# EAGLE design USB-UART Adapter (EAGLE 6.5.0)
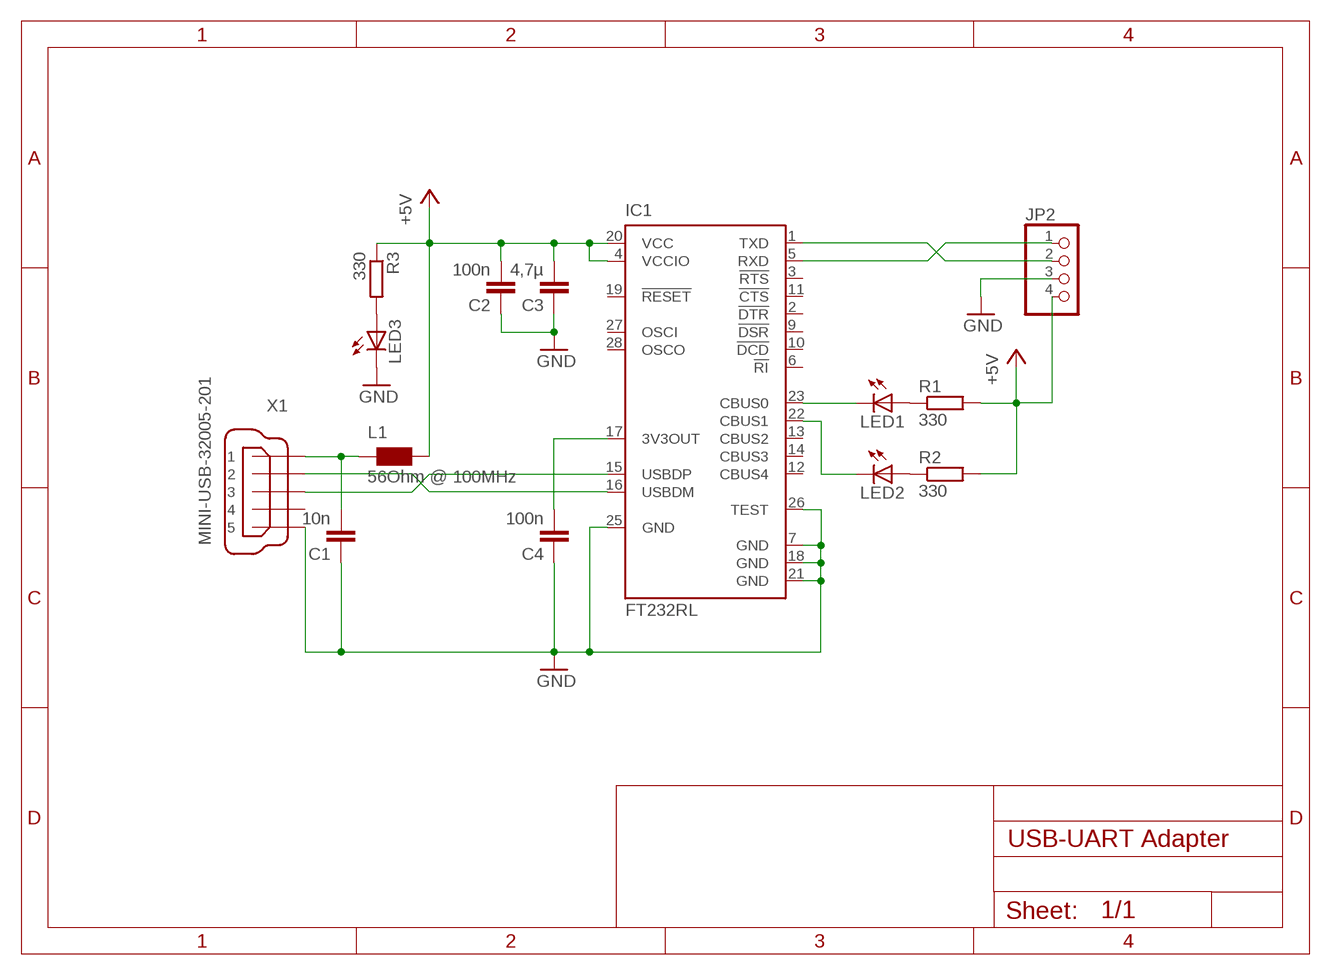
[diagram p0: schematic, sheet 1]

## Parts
C1  10n  C-EUC0805  [C0805]
C2  100n  C-EUC0805  [C0805]
C3  4,7µ  C-EUC0805  [C0805]
C4  100n  C-EUC0805  [C0805]
IC1  FT232RL  [SSOP28]
JP2  PINHD-1X4  [1X04]
L1  56Ohm @ 100MHz  SMD_BEADS_FASTRON_SMB/001  [SMB/001]
LED1  LEDSML0805  [SML0805]
LED2  LEDSML0805  [SML0805]
LED3  LEDSML0805  [SML0805]
R1  330  R-EU_R0805  [R0805]
R2  330  R-EU_R0805  [R0805]
R3  330  R-EU_R0805  [R0805]
X1  MINI-USB-32005-201  [32005-201]

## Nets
+5V: C2.2 C3.2 IC1.4(VCCIO) IC1.20(VCC) JP2.4 L1.2 R1.2 R2.2 R3.1
GND: C1.1 C2.1 C3.1 C4.1 IC1.7(GND) IC1.18(GND) IC1.21(GND) IC1.25(GND) IC1.26(TEST) JP2.3 LED3.C X1.5
N$1: IC1.5(RXD) JP2.1
N$2: IC1.1(TXD) JP2.2
N$3: IC1.16(USBDM) X1.2
N$4: IC1.23(CBUS0) LED1.C
N$5: C4.2 IC1.17(3V3OUT)
N$6: IC1.15(USBDP) X1.3
N$7: IC1.22(CBUS1) LED2.C
N$8: LED1.A R1.1
N$9: C1.2 L1.1 X1.1
N$12: LED2.A R2.1
N$14: LED3.A R3.2
Unconnected: IC1.2(!DTR) IC1.3(!RTS) IC1.6(!RI) IC1.9(!DSR) IC1.10(!DCD) IC1.11(!CTS) IC1.12(CBUS4) IC1.13(CBUS2) IC1.14(CBUS3) IC1.19(!RESET) IC1.27(OSCI) IC1.28(OSCO) X1.4

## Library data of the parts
C1-C4 = rcl:C-EU: CAPACITOR, European symbol
IC1 = ftdichip:FT232R: Source: http://www.ftdichip.com/Documents/DataSheets/DS_FT232R_v104.pdf; MPN: FT232RL; OC_FARNELL: 1146032; OC_NEWARK: 91K9918
JP2 = pinhead:PINHD-1X4: PIN HEADER
L1 = eigene:SMD_BEADS_FASTRON: SMD EMI Suppression Ferrite Beads
LED1-LED3 = led:LED: LED
R1-R3 = rcl:R-EU_: RESISTOR, European symbol
X1 = con-cypressindustries:MINI-USB-: MINI USB-B Conector Source: www.cypressindustries.com; OC_FARNELL: unknown; OC_NEWARK: unknown

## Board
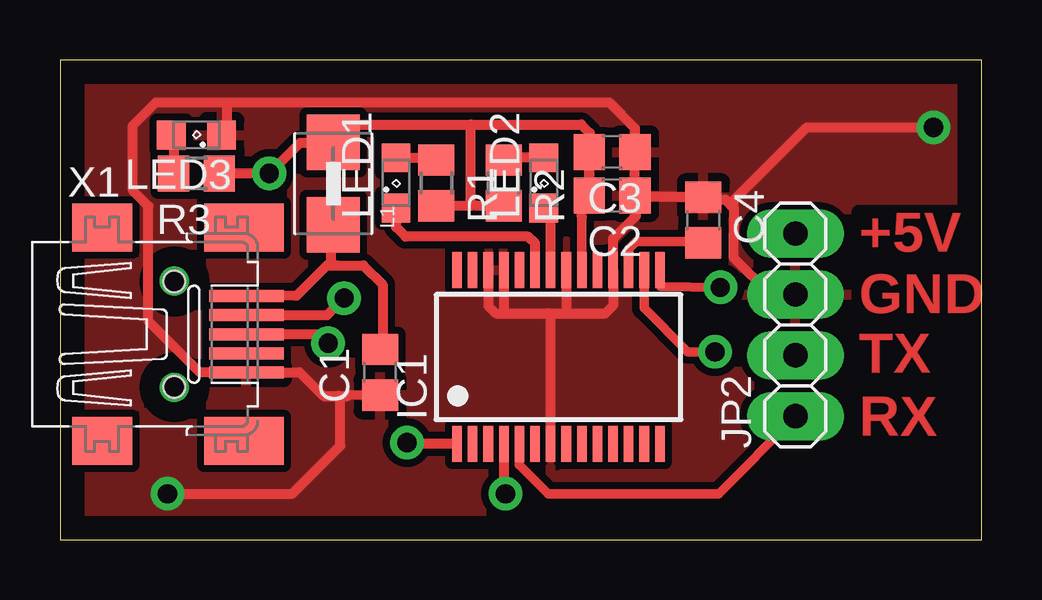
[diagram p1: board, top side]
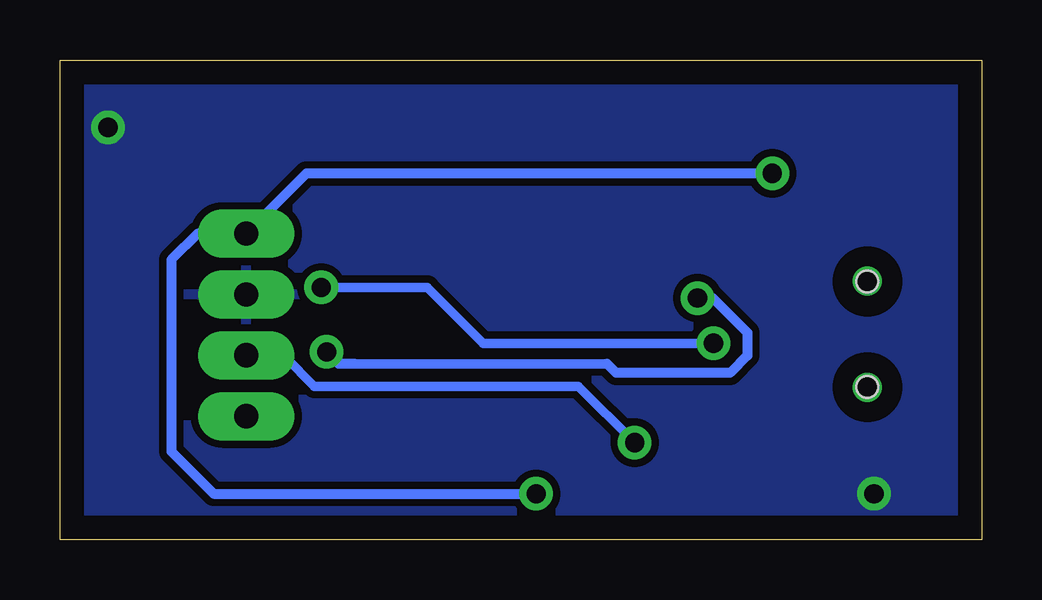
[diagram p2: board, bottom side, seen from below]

Size 38.4 x 20.01 mm. Coordinates in mm from the lower left corner, seen from the top.
Outline: 0,0 38.4,0 38.4,20.01 0,20.01 0,0
Copper layers (1*16): Top 0.035mm / dielectric 1.5mm / Bottom 0.035mm
Design rules "SMD_zweiseitig": minimum track width 0.3mm, minimum drill 0.8mm, track to track 0.2mm, track to pad 0.2mm, pad to pad 0.2mm, via to via 0.2mm, smd to smd 0.2mm, copper to edge 1mm, drill to drill 1mm, minimum pad ring 0.5mm, minimum via ring 0.3mm, stop-mask expansion 4mil, vias tented up to drill 0mil, thermal gap 14mil

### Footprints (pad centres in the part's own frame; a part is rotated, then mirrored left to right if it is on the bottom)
C0805 = smd 1.3 x 1.5: 1 -0.95,0; 2 0.95,0
SSOP28 = smd 0.4 x 1.5: 1 -4.225,-3.625; 2 -3.575,-3.625; 3 -2.925,-3.625; 4 -2.275,-3.625; 5 -1.625,-3.625; 6 -0.975,-3.625; 7 -0.325,-3.625; 8 0.325,-3.625; 9 0.975,-3.625; 10 1.625,-3.625; 11 2.275,-3.625; 12 2.925,-3.625; 13 3.575,-3.625; 14 4.225,-3.625; 15 4.225,3.625; 16 3.575,3.625; 17 2.925,3.625; 18 2.275,3.625; 19 1.625,3.625; 20 0.975,3.625; 21 0.325,3.625; 22 -0.325,3.625; 23 -0.975,3.625; 24 -1.625,3.625; 25 -2.275,3.625; 26 -2.925,3.625; 27 -3.575,3.625; 28 -4.225,3.625
1X04 = drill 1.016 long: 1 -3.81,0; 2 -1.27,0; 3 1.27,0; 4 3.81,0
SMB/001 = smd 2.3 x 2.2: 1 -1.72,0; 2 1.72,0
SML0805 = smd 1.2 x 1.2: A 1.05,0; C -1.05,0
R0805 = smd 1.3 x 1.5: 1 -0.95,0; 2 0.95,0
32005-201 = smd 3.1 x 0.5: 1 3,1.6; 2 3,0.8; 3 3,0; 4 3,-0.8; 5 3,-1.6 | smd 2.5 x 2: M1 -3,-4.45; M2 -3,4.45 | smd 3.3 x 2: M3 2.9,4.45; M4 2.9,-4.45 | hole 0.9: 0,2.2; 0,-2.2

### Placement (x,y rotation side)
C1  13.34,6.99 90 top
C2  23,14.36 180 top
C3  23,16.18 180 top
C4  26.8,13.34 270 top
IC1  20.77,7.62 0 top
JP2  30.64,8.96 90 top
L1  11.39,14.86 90 top
LED1  14,14.88 90 top
LED2  20.16,14.88 90 top
LED3  5.68,16.88 180 top
R1  15.68,14.88 270 top
R2  18.48,14.88 270 top
R3  5.68,15.28 180 top
X1  4.76,8.57 0 top

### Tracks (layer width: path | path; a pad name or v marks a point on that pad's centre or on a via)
+5V  (via drill 0.8)
  Top 0.4: 21.74,13.46 IC1.20
  Top 0.406: IC1.4 18.5,1.99 v18.56,1.92 | 21.74,13.46 21.74,14.04 C2.2 | C2.2 C3.2 | R1.2 17.12,13.93 | R2.2 17.36,13.93 17.12,13.93 | C2.2 22.08,14.38 22.08,16.96 21.72,17.32 17.12,17.32 | 17.12,17.32 11.65,17.32 L1.2 11.37,16.56 10,16.56 v8.72,15.28 R3.1 | 17.12,13.93 17.12,17.32
  Bottom 0.406: v18.56,1.92 32,1.92 33.76,3.68 33.76,11.68 32.67,12.77 JP2.4 28.13,15.28 v8.72,15.28
GND  (via drill 0.8)
  Top 0.4: IC1.7 | 7.82,6.98 7.78,6.98 X1.5 | 12.06,6.04 C1.1 13.52,6.12 | C4.1 26.98,14.18
  Top 0.406: IC1.26 17.84,9.76 18.16,9.44 18.56,9.44 | 18.56,9.44 20.32,9.44 | 20.32,9.44 21.12,9.44 | 21.12,9.44 22.72,9.44 23.05,9.77 IC1.18 23.05,12.56 24,13.52 24,14.31 C2.1 | IC1.21 21.09,9.46 21.12,9.44 | IC1.25 18.5,9.51 18.56,9.44 | IC1.7 20.45,9.31 20.32,9.44 | 6.96,18.24 4,18.24 3.04,17.28 3.04,14.56 3.68,13.92 3.68,9.12 5.82,6.98 7.82,6.98 9.98,6.98 10.96,6 11.6,6 | 6.96,18.24 22.88,18.24 23.95,17.16 C3.1 C2.1 | 11.6,6 12.02,6 12.06,6.04 | 26.98,14.18 27.74,14.18 28.08,13.84 | 28.08,13.84 28.06,11.78 29.6,10.24 JP2.3 | C4.1 24.03,14.29 C2.1 | LED3.C 6.96,17.11 6.96,18.24 | v4.48,1.92 9.68,1.92 11.68,3.92 11.68,5.92 11.6,6 | 28.08,13.84 28.08,14.16 31.12,17.2 v36.4,17.2
  pour Top (isolate 0.305): 0.08,-0.08 38.48,-0.08 38.4,19.92 0,19.92
  pour Bottom (isolate 0.305): 0,0 0,19.92 38.48,19.92 38.48,0
N$1
  Top 0.4: 30.6,5.08 27.44,1.92 20.34,1.92 19.14,3.12 19.14,3.98 IC1.5
  Top 0.406: 30.6,5.08 30.6,5.11 JP2.1
N$2  (via drill 0.8)
  Top 0.4: IC1.1
  Top 0.406: IC1.1 14.51,4 v14.46,4.05
  Bottom 0.4: v14.46,4.05 16.81,6.41 27.8,6.41 29.01,7.62
  Bottom 0.406: 29.01,7.62 30.57,7.62 JP2.2
N$3  (via drill 0.8)
  Top 0.4: v27.29,7.84 26.16,7.84 24.34,9.66 IC1.16
  Top 0.406: X1.2 11.13,9.37 v11.84,10.08
  Bottom 0.4: 15.6,7.34 26.12,7.34
  Bottom 0.406: v11.84,10.08 11.2,10.08 9.76,8.64 9.76,7.68 10.48,6.96 15.22,6.96 15.6,7.34 | 26.12,7.34 26.79,7.34 v27.29,7.84
N$4
  Top 0.406: IC1.23 19.8,12.37 19.52,12.64 14.4,12.64 14,13.04 LED1.C
N$5
  Top 0.4: IC1.17 23.7,12.12 24.02,12.44 26.7,12.44 26.76,12.38 C4.2
N$6  (via drill 0.8)
  Top 0.4: v27.52,10.53 25.04,10.56 25,10.6 IC1.15 | X1.3 7.78,8.58
  Top 0.406: 7.78,8.58 10.79,8.58 v11.17,8.2
  Bottom 0.4: v27.52,10.53 23.1,10.53 20.77,8.2 v11.17,8.2
N$7
  Top 0.406: IC1.22 20.45,13.54 LED2.C
N$8
  Top 0.406: LED1.A 15.22,15.93 R1.1
N$9
  Top 0.4: 13.71,7.94 13.32,7.94 C1.2 | 9.79,10.18 7.78,10.18 X1.1 | 11.66,13.64 L1.1
  Top 0.406: 13.36,7.96 C1.2 13.44,8.04 13.44,10.64 12.64,11.44 11.52,11.44 | 9.79,10.18 9.86,10.18 11.12,11.44 11.28,11.44 | 11.28,11.44 11.52,11.44 | 11.54,11.46 11.52,11.44 | L1.1 11.28,13.13 11.28,11.44
N$10  (via drill 0.6)
  other vias: 4.76,10.79
N$11  (via drill 0.6)
  other vias: 4.76,6.35
N$12
  Top 0.406: LED2.A 18.58,15.93 R2.1
N$14
  Top 0.406: LED3.A 4.73,16.78 R3.2

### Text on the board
Top: +5V | GND | TX | RX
